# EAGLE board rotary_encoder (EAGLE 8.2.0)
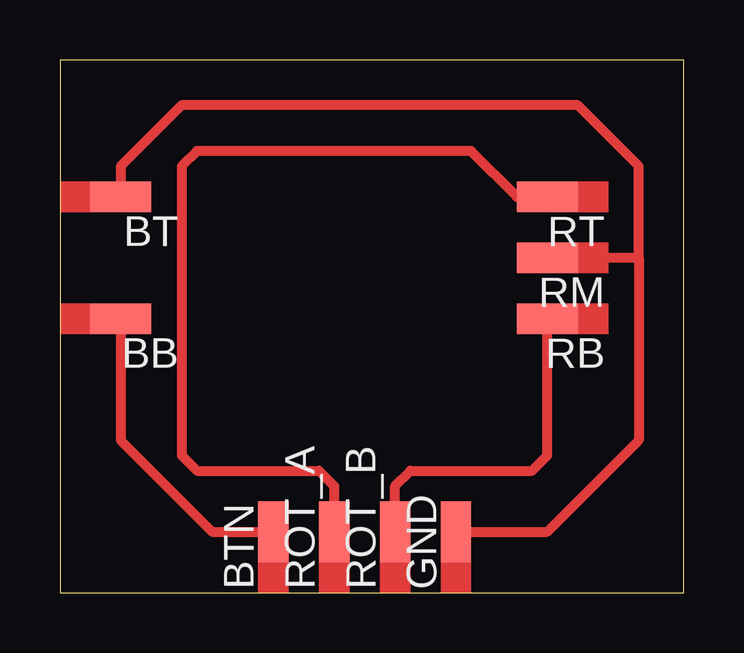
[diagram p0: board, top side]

Size 26.02 x 22.21 mm. Coordinates in mm from the lower left corner, seen from the top.
Outline: 0,0 26.02,0 26.02,22.21 0,22.21 0,0
Copper layers (1*16): Top 0.035mm / dielectric 1.5mm / Bottom 0.035mm
Design rules "default *": minimum track width 10mil, minimum drill 24mil, track to track 16mil, track to pad 16mil, pad to pad 16mil, via to via 16mil, smd to smd 16mil, copper to edge 40mil, drill to drill 8mil, minimum pad ring 10mil, minimum via ring 8mil, stop-mask expansion 4mil, vias tented up to drill 0mil, thermal gap 10mil

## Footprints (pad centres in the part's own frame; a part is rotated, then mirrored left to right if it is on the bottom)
SMD1,27-2,54 = smd 1.27 x 2.54: 1 0,0

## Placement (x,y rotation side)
BB  [SMD1,27-2,54]  2.54,11.43 90 top
BT  [SMD1,27-2,54]  2.54,16.51 90 top
BTN  [SMD1,27-2,54]  8.89,2.54 0 top
GND  [SMD1,27-2,54]  16.51,2.54 0 top
RB  [SMD1,27-2,54]  20.32,11.43 90 top
RM  [SMD1,27-2,54]  20.32,13.97 90 top
ROT_A  [SMD1,27-2,54]  11.43,2.54 0 top
ROT_B  [SMD1,27-2,54]  13.97,2.54 0 top
RT  [SMD1,27-2,54]  20.32,16.51 90 top

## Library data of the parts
BB BT BTN GND RB RM ROT_A ROT_B RT = wirepad

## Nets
GND: BT.1 GND.1 RM.1
PIN_A: ROT_A.1 RT.1
PIN_B: RB.1 ROT_B.1
SWITCH: BB.1 BTN.1

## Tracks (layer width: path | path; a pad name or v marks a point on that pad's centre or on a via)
GND
  Top 0.406: GND.1 20.32,2.54 24.13,6.35 24.13,13.97 | 24.13,13.97 24.13,17.78 21.59,20.32 5.08,20.32 2.54,17.78 BT.1 | RM.1 24.13,13.97
PIN_A
  Top 0.406: RT.1 19.05,16.51 17.14,18.41 5.71,18.41 5.08,17.78 5.08,5.71 5.71,5.08 10.79,5.08 11.43,4.45 ROT_A.1
PIN_B
  Top 0.406: ROT_B.1 13.97,4.45 14.61,5.08 19.68,5.08 20.32,5.71 RB.1
SWITCH
  Top 0.406: BB.1 2.54,6.35 6.35,2.54 BTN.1
(copper drawn outside any net)
  shapes: Top area x9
